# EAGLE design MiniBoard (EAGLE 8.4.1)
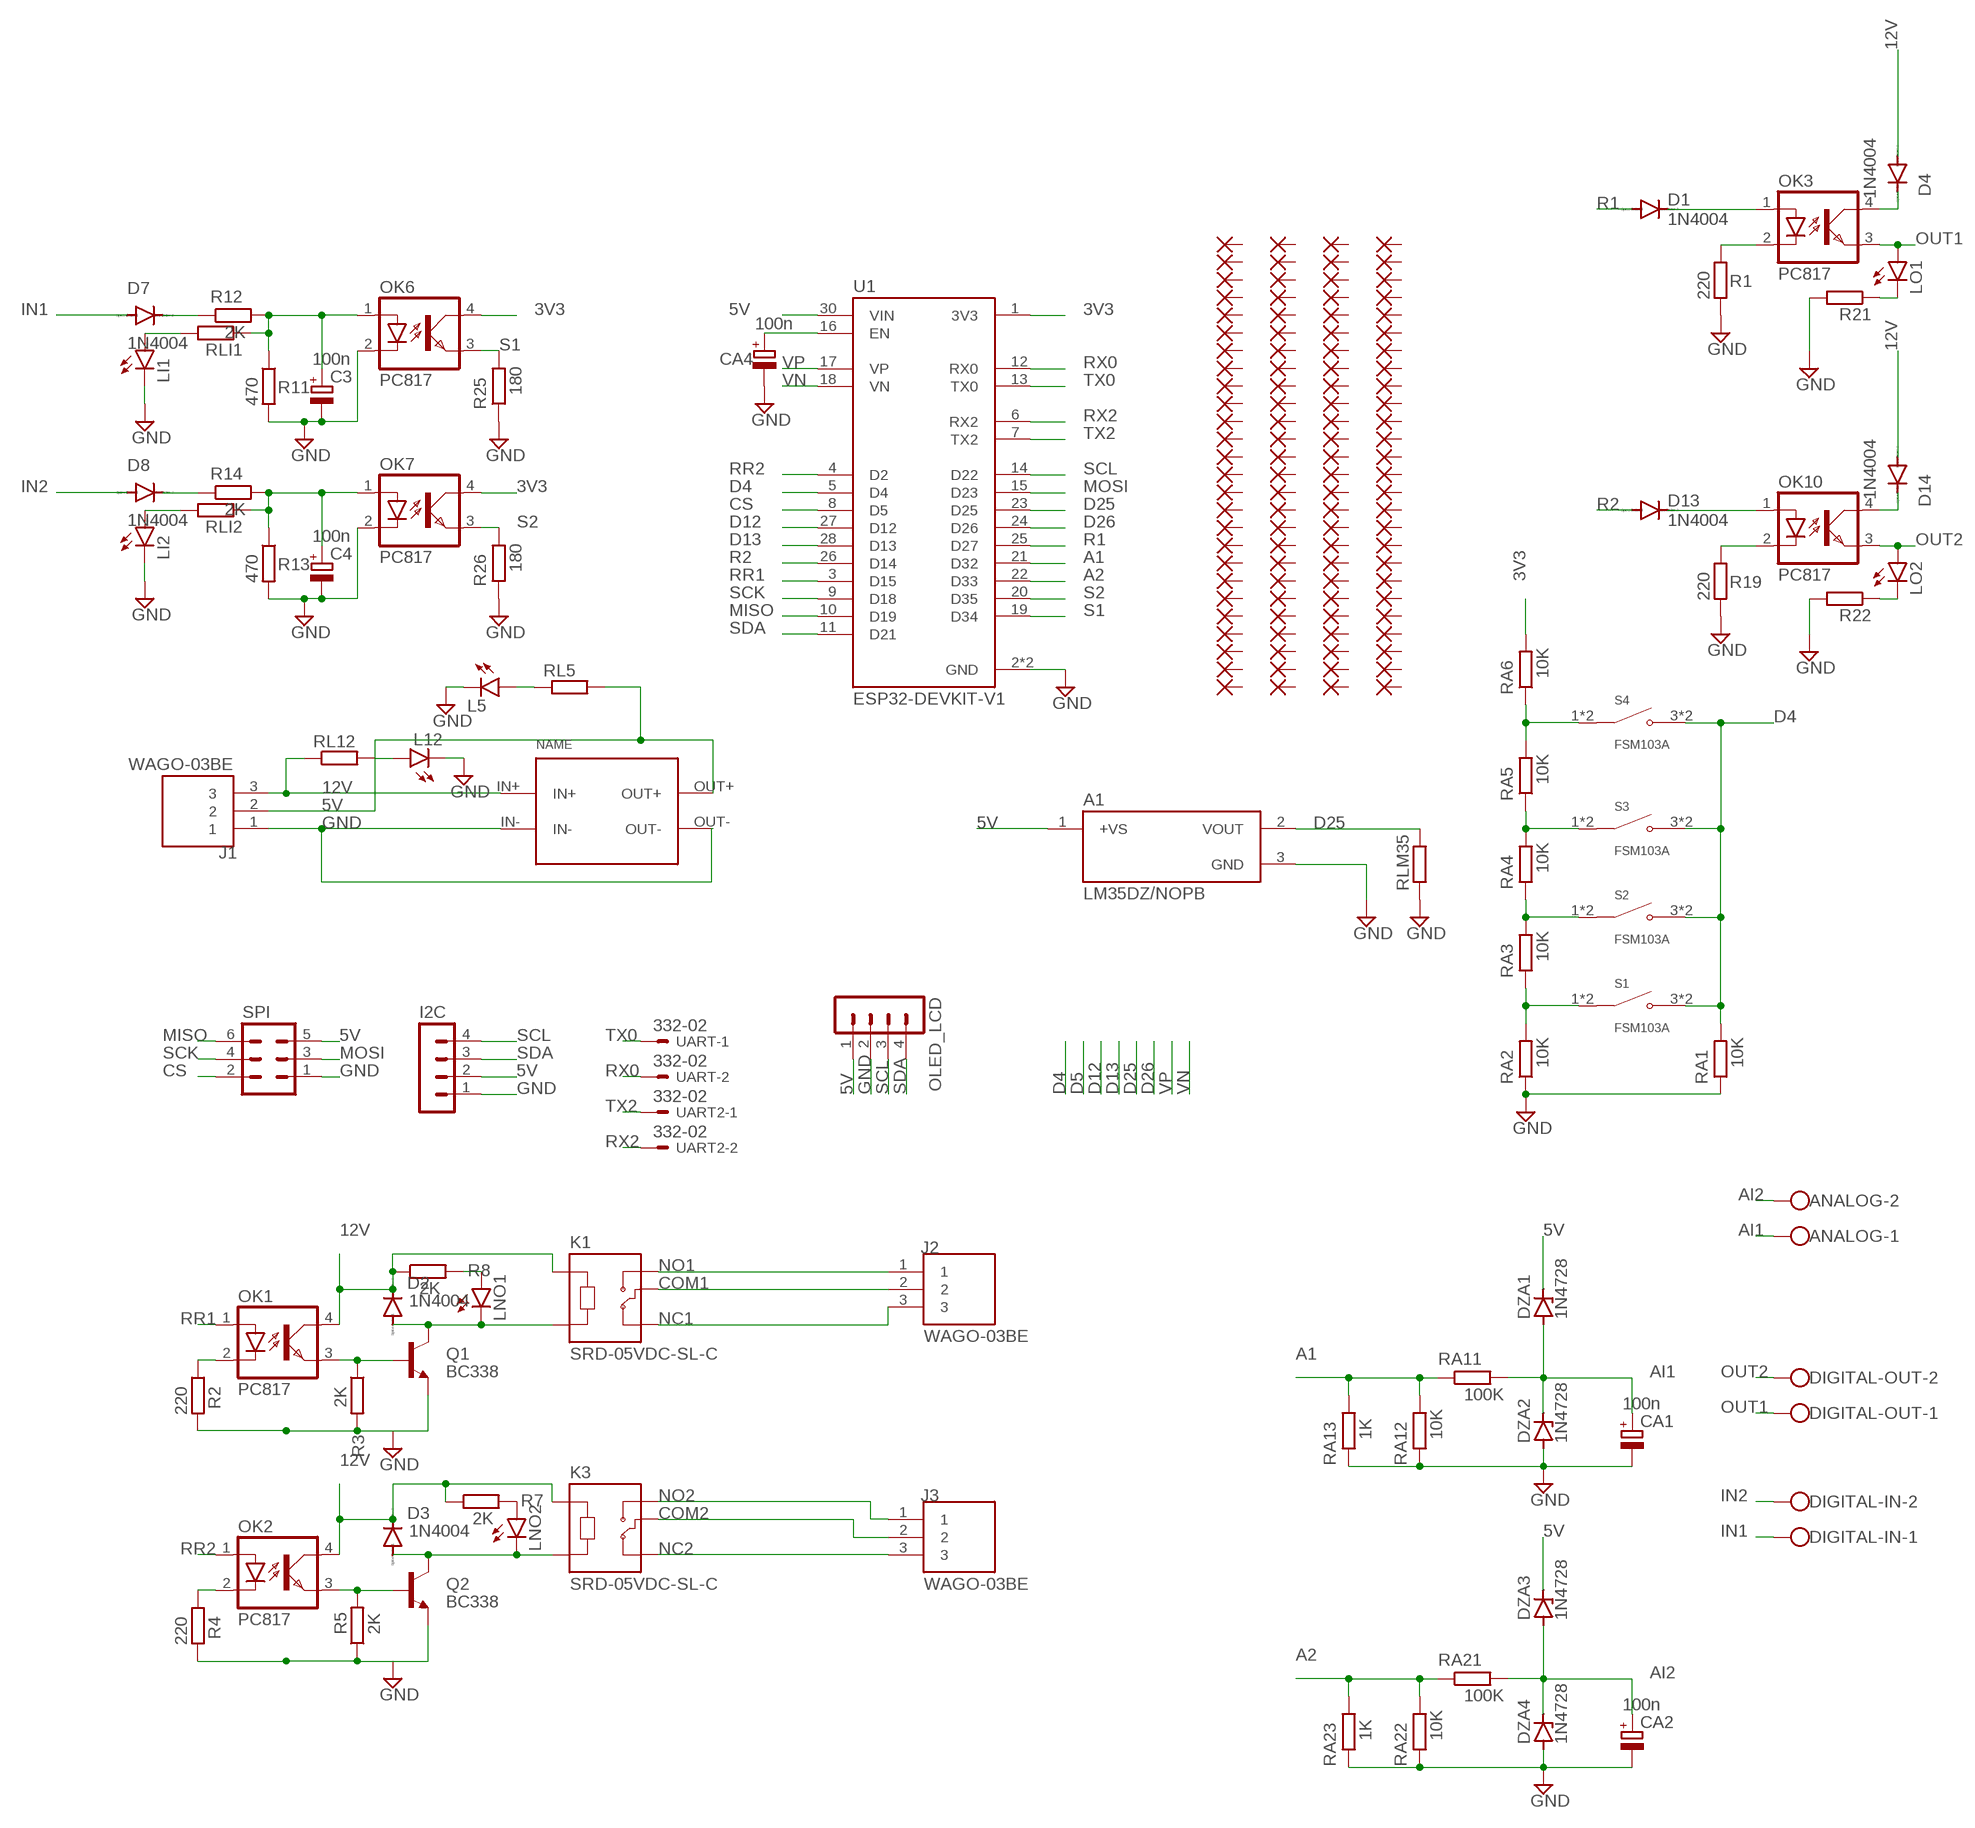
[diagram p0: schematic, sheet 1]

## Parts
A1  LM35DZ/NOPB  [TO92127P521H735-3]
ANALOG  W237-102  [W237-102]
C3  100n  CPOL-EUE5-6  [E5-6]
C4  100n  CPOL-EUE5-6  [E5-6]
CA1  100n  CPOL-EUE5-6  [E5-6]
CA2  100n  CPOL-EUE5-6  [E5-6]
CA4  100n  CPOL-EUE5-6  [E5-6]
D1  1N4004  [DO41-10]
D2  1N4004  [DO41-10]
D3  1N4004  [DO41-10]
D4  1N4004  [DO41-10]
D7  1N4004  [DO41-10]
D8  1N4004  [DO41-10]
D13  1N4004  [DO41-10]
D14  1N4004  [DO41-10]
DIGITAL-IN  W237-102  [W237-102]
DIGITAL-OUT  W237-102  [W237-102]
DZA1  1N4728  [DO41Z10]
DZA2  1N4728  [DO41Z10]
DZA3  1N4728  [DO41Z10]
DZA4  1N4728  [DO41Z10]
I2C  MA04-1  [MA04-1]
J1  WAGO-03BE  [CUI_TB006-508-03BE]
J2  WAGO-03BE  [CUI_TB006-508-03BE]
J3  WAGO-03BE  [CUI_TB006-508-03BE]
K1  SRD-05VDC-SL-C  [RELAY_SRD-05VDC-SL-C]
K3  SRD-05VDC-SL-C  [RELAY_SRD-05VDC-SL-C]
L5  LED3MM  [LED3MM]
L12  LED3MM  [LED3MM]
LI1  LED3MM  [LED3MM]
LI2  LED3MM  [LED3MM]
LNO1  LED3MM  [LED3MM]
LNO2  LED3MM  [LED3MM]
LO1  LED3MM  [LED3MM]
LO2  LED3MM  [LED3MM]
OK1  PC817  [DIL04]
OK2  PC817  [DIL04]
OK3  PC817  [DIL04]
OK6  PC817  [DIL04]
OK7  PC817  [DIL04]
OK10  PC817  [DIL04]
OLED_LCD  MA04-1  [MA04-1]
PAD1  WIREPAD1,6/0,9  [1,6/0,9]
PAD2  WIREPAD1,6/0,9  [1,6/0,9]
PAD3  WIREPAD1,6/0,9  [1,6/0,9]
PAD4  WIREPAD1,6/0,9  [1,6/0,9]
PAD5  WIREPAD1,6/0,9  [1,6/0,9]
PAD6  WIREPAD1,6/0,9  [1,6/0,9]
PAD7  WIREPAD1,6/0,9  [1,6/0,9]
PAD8  WIREPAD1,6/0,9  [1,6/0,9]
PAD9  WIREPAD1,6/0,9  [1,6/0,9]
PAD10  WIREPAD1,6/0,9  [1,6/0,9]
PAD11  WIREPAD1,6/0,9  [1,6/0,9]
PAD12  WIREPAD1,6/0,9  [1,6/0,9]
PAD13  WIREPAD1,6/0,9  [1,6/0,9]
PAD14  WIREPAD1,6/0,9  [1,6/0,9]
PAD15  WIREPAD1,6/0,9  [1,6/0,9]
PAD16  WIREPAD1,6/0,9  [1,6/0,9]
PAD17  WIREPAD1,6/0,9  [1,6/0,9]
PAD18  WIREPAD1,6/0,9  [1,6/0,9]
PAD19  WIREPAD1,6/0,9  [1,6/0,9]
PAD20  WIREPAD1,6/0,9  [1,6/0,9]
PAD21  WIREPAD1,6/0,9  [1,6/0,9]
PAD22  WIREPAD1,6/0,9  [1,6/0,9]
PAD23  WIREPAD1,6/0,9  [1,6/0,9]
PAD24  WIREPAD1,6/0,9  [1,6/0,9]
PAD25  WIREPAD1,6/0,9  [1,6/0,9]
PAD26  WIREPAD1,6/0,9  [1,6/0,9]
PAD27  WIREPAD1,6/0,9  [1,6/0,9]
PAD28  WIREPAD1,6/0,9  [1,6/0,9]
PAD29  WIREPAD1,6/0,9  [1,6/0,9]
PAD30  WIREPAD1,6/0,9  [1,6/0,9]
PAD31  WIREPAD1,6/0,9  [1,6/0,9]
PAD32  WIREPAD1,6/0,9  [1,6/0,9]
PAD33  WIREPAD1,6/0,9  [1,6/0,9]
PAD34  WIREPAD1,6/0,9  [1,6/0,9]
PAD35  WIREPAD1,6/0,9  [1,6/0,9]
PAD36  WIREPAD1,6/0,9  [1,6/0,9]
PAD37  WIREPAD1,6/0,9  [1,6/0,9]
PAD38  WIREPAD1,6/0,9  [1,6/0,9]
PAD39  WIREPAD1,6/0,9  [1,6/0,9]
PAD40  WIREPAD1,6/0,9  [1,6/0,9]
PAD41  WIREPAD1,6/0,9  [1,6/0,9]
PAD42  WIREPAD1,6/0,9  [1,6/0,9]
PAD43  WIREPAD1,6/0,9  [1,6/0,9]
PAD44  WIREPAD1,6/0,9  [1,6/0,9]
PAD45  WIREPAD1,6/0,9  [1,6/0,9]
PAD46  WIREPAD1,6/0,9  [1,6/0,9]
PAD47  WIREPAD1,6/0,9  [1,6/0,9]
PAD48  WIREPAD1,6/0,9  [1,6/0,9]
PAD49  WIREPAD1,6/0,9  [1,6/0,9]
PAD50  WIREPAD1,6/0,9  [1,6/0,9]
PAD51  WIREPAD1,6/0,9  [1,6/0,9]
PAD52  WIREPAD1,6/0,9  [1,6/0,9]
PAD53  WIREPAD1,6/0,9  [1,6/0,9]
PAD54  WIREPAD1,6/0,9  [1,6/0,9]
PAD55  WIREPAD1,6/0,9  [1,6/0,9]
PAD56  WIREPAD1,6/0,9  [1,6/0,9]
PAD57  WIREPAD1,6/0,9  [1,6/0,9]
PAD58  WIREPAD1,6/0,9  [1,6/0,9]
PAD59  WIREPAD1,6/0,9  [1,6/0,9]
PAD60  WIREPAD1,6/0,9  [1,6/0,9]
PAD61  WIREPAD1,6/0,9  [1,6/0,9]
PAD62  WIREPAD1,6/0,9  [1,6/0,9]
PAD63  WIREPAD1,6/0,9  [1,6/0,9]
PAD64  WIREPAD1,6/0,9  [1,6/0,9]
PAD65  WIREPAD1,6/0,9  [1,6/0,9]
PAD66  WIREPAD1,6/0,9  [1,6/0,9]
PAD67  WIREPAD1,6/0,9  [1,6/0,9]
PAD68  WIREPAD1,6/0,9  [1,6/0,9]
PAD69  WIREPAD1,6/0,9  [1,6/0,9]
PAD70  WIREPAD1,6/0,9  [1,6/0,9]
PAD71  WIREPAD1,6/0,9  [1,6/0,9]
PAD72  WIREPAD1,6/0,9  [1,6/0,9]
PAD73  WIREPAD1,6/0,9  [1,6/0,9]
PAD74  WIREPAD1,6/0,9  [1,6/0,9]
PAD75  WIREPAD1,6/0,9  [1,6/0,9]
PAD76  WIREPAD1,6/0,9  [1,6/0,9]
PAD77  WIREPAD1,6/0,9  [1,6/0,9]
PAD78  WIREPAD1,6/0,9  [1,6/0,9]
PAD79  WIREPAD1,6/0,9  [1,6/0,9]
PAD80  WIREPAD1,6/0,9  [1,6/0,9]
PAD81  WIREPAD1,6/0,9  [1,6/0,9]
PAD82  WIREPAD1,6/0,9  [1,6/0,9]
PAD83  WIREPAD1,6/0,9  [1,6/0,9]
PAD84  WIREPAD1,6/0,9  [1,6/0,9]
PAD85  WIREPAD1,6/0,9  [1,6/0,9]
PAD86  WIREPAD1,6/0,9  [1,6/0,9]
PAD87  WIREPAD1,6/0,9  [1,6/0,9]
PAD88  WIREPAD1,6/0,9  [1,6/0,9]
PAD89  WIREPAD1,6/0,9  [1,6/0,9]
PAD90  WIREPAD1,6/0,9  [1,6/0,9]
PAD91  WIREPAD1,6/0,9  [1,6/0,9]
PAD92  WIREPAD1,6/0,9  [1,6/0,9]
PAD93  WIREPAD1,6/0,9  [1,6/0,9]
PAD94  WIREPAD1,6/0,9  [1,6/0,9]
PAD95  WIREPAD1,6/0,9  [1,6/0,9]
PAD96  WIREPAD1,6/0,9  [1,6/0,9]
PAD97  WIREPAD1,6/0,9  [1,6/0,9]
PAD98  WIREPAD1,6/0,9  [1,6/0,9]
PAD99  WIREPAD1,6/0,9  [1,6/0,9]
PAD100  WIREPAD1,6/0,9  [1,6/0,9]
PAD101  WIREPAD1,6/0,9  [1,6/0,9]
PAD102  WIREPAD1,6/0,9  [1,6/0,9]
PAD103  WIREPAD1,6/0,9  [1,6/0,9]
PAD104  WIREPAD1,6/0,9  [1,6/0,9]
Q1  BC338  [TO92-EBC]
Q2  BC338  [TO92-EBC]
R1  220  R-EU_0309/12  [0309/12]
R2  220  R-EU_0309/12  [0309/12]
R3  2K  R-EU_0309/12  [0309/12]
R4  220  R-EU_0309/12  [0309/12]
R5  2K  R-EU_0309/12  [0309/12]
R7  2K  R-EU_0309/12  [0309/12]
R8  2K  R-EU_0309/12  [0309/12]
R11  470  R-EU_0309/12  [0309/12]
R12  2K  R-EU_0309/12  [0309/12]
R13  470  R-EU_0309/12  [0309/12]
R14  2K  R-EU_0309/12  [0309/12]
R19  220  R-EU_0309/12  [0309/12]
R21  R-EU_0309/12  [0309/12]
R22  R-EU_0309/12  [0309/12]
R25  180  R-EU_0309/12  [0309/12]
R26  180  R-EU_0309/12  [0309/12]
RA1  10K  R-EU_0309/12  [0309/12]
RA2  10K  R-EU_0309/12  [0309/12]
RA3  10K  R-EU_0309/12  [0309/12]
RA4  10K  R-EU_0309/12  [0309/12]
RA5  10K  R-EU_0309/12  [0309/12]
RA6  10K  R-EU_0309/12  [0309/12]
RA11  100K  R-EU_0309/12  [0309/12]
RA12  10K  R-EU_0309/12  [0309/12]
RA13  1K  R-EU_0309/12  [0309/12]
RA21  100K  R-EU_0309/12  [0309/12]
RA22  10K  R-EU_0309/12  [0309/12]
RA23  1K  R-EU_0309/12  [0309/12]
RL5  R-EU_0309/12  [0309/12]
RL12  R-EU_0309/12  [0309/12]
RLI1  R-EU_0309/12  [0309/12]
RLI2  R-EU_0309/12  [0309/12]
RLM35  R-EU_0309/12  [0309/12]
S1  FSM103A  [SW_1571627-1]
S2  FSM103A  [SW_1571627-1]
S3  FSM103A  [SW_1571627-1]
S4  FSM103A  [SW_1571627-1]
SPI  MA03-2  [MA03-2]
U1  ESP32-DEVKIT-V1  [MODULE_ESP32_DEVKIT_V1]
U$1  CP8-ADJ  [CP8-ADJ]
UART  332-02  [332-02]
UART2  332-02  [332-02]

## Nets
3V3: OK6.4(COL) OK7.4(COL) RA6.2 U1.1(3V3)
5V: A1.1(+VS) DZA1.C DZA3.C I2C.2 J1.2 OLED_LCD.1 RL5.2 SPI.5 U1.30(VIN) U$1.OUT+
12V: D2.C D3.C D4.A D14.A J1.3 K1.A1 K3.A1 OK1.4(COL) OK2.4(COL) R7.1 R8.1 RL12.1 U$1.IN+
A1: RA11.1 RA12.2 RA13.2 U1.21(D32)
A2: RA21.1 RA22.2 RA23.2 U1.22(D33)
AI1: ANALOG.1 CA1.+ DZA1.A DZA2.C RA11.2
AI2: ANALOG.2 CA2.+ DZA3.A DZA4.C RA21.2
COM1: J2.2 K1.COM
COM2: J3.2 K3.COM
CS: SPI.2 U1.8(D5)
D4: RA1.2 S1.3(NO) S1.4(NO) S2.3(NO) S2.4(NO) S3.3(NO) S3.4(NO) S4.3(NO) S4.4(NO) U1.5(D4)
D12: U1.27(D12)
D13: U1.28(D13)
D25: A1.2(VOUT) RLM35.2 U1.23(D25)
D26: U1.24(D26)
GND: A1.3(GND) C3.- C4.- CA1.- CA2.- CA4.- DZA2.A DZA4.A I2C.1 J1.1 L5.K(C) L12.K(C) LI1.K(C) LI2.K(C) OK6.2(C) OK7.2(C) OLED_LCD.2 Q1.E Q2.E R1.2 R2.2 R3.2 R4.2 R5.1 R11.2 R13.2 R19.2 R21.2 R22.2 R25.1 R26.1 RA1.1 RA2.1 RA12.1 RA13.1 RA22.1 RA23.1 RLM35.1 SPI.1 U1.2(GND) U1.29(GND) U$1.IN- U$1.OUT-
IN1: D7.A DIGITAL-IN.1
IN2: D8.A DIGITAL-IN.2
MISO: SPI.6 U1.10(D19)
MOSI: SPI.3 U1.15(D23)
N$1: OK2.2(C) R4.1
N$2: OK1.2(C) R2.1
N$3: OK1.3(EMIT) Q1.B R3.1
N$4: D3.A K3.A2 LNO2.K(C) Q2.C
N$5: RA4.2 RA5.1 S3.1(COM) S3.2(COM)
N$6: OK2.3(EMIT) Q2.B R5.2
N$7: LNO2.A R7.2
N$8: RA3.2 RA4.1 S2.1(COM) S2.2(COM)
N$9: RA2.2 RA3.1 S1.1(COM) S1.2(COM)
N$10: LNO1.A R8.2
N$11: D2.A K1.A2 LNO1.K(C) Q1.C
N$14: L12.A RL12.2
N$15: D1.C OK3.1(A)
N$16: OK3.2(C) R1.1
N$18: D4.C OK3.4(COL)
N$19: C3.+ OK6.1(A) R11.1 R12.2 RLI1.1
N$20: D7.C R12.1
N$21: C4.+ OK7.1(A) R13.1 R14.2 RLI2.1
N$22: D8.C R14.1
N$23: L5.A RL5.1
N$24: LI2.A RLI2.2
N$25: CA4.+ U1.16(EN)
N$26: D13.C OK10.1(A)
N$27: OK10.2(C) R19.1
N$29: LI1.A RLI1.2
N$30: LO1.K(C) R21.1
N$31: LO2.K(C) R22.1
N$32: RA5.2 RA6.1 S4.1(COM) S4.2(COM)
N$52: D14.C OK10.4(COL)
NC1: J2.3 K1.NC
NC2: J3.3 K3.NC
NO1: J2.1 K1.NO
NO2: J3.1 K3.NO
OUT1: DIGITAL-OUT.1 LO1.A OK3.3(EMIT)
OUT2: DIGITAL-OUT.2 LO2.A OK10.3(EMIT)
R1: D1.A U1.25(D27)
R2: D13.A U1.26(D14)
RR1: OK1.1(A) U1.3(D15)
RR2: OK2.1(A) U1.4(D2)
RX0: U1.12(RX0) UART.2
RX2: U1.6(RX2) UART2.2
S1: OK6.3(EMIT) R25.2 U1.19(D34)
S2: OK7.3(EMIT) R26.2 U1.20(D35)
SCK: SPI.4 U1.9(D18)
SCL: I2C.4 OLED_LCD.3 U1.14(D22)
SDA: I2C.3 OLED_LCD.4 U1.11(D21)
TX0: U1.13(TX0) UART.1
TX2: U1.7(TX2) UART2.1
VN: U1.18(VN)
VP: U1.17(VP)
Unconnected: PAD1.1(P) PAD2.1(P) PAD3.1(P) PAD4.1(P) PAD5.1(P) PAD6.1(P) PAD7.1(P) PAD8.1(P) PAD9.1(P) PAD10.1(P) PAD11.1(P) PAD12.1(P) PAD13.1(P) PAD14.1(P) PAD15.1(P) PAD16.1(P) PAD17.1(P) PAD18.1(P) PAD19.1(P) PAD20.1(P) PAD21.1(P) PAD22.1(P) PAD23.1(P) PAD24.1(P) PAD25.1(P) PAD26.1(P) PAD27.1(P) PAD28.1(P) PAD29.1(P) PAD30.1(P) PAD31.1(P) PAD32.1(P) PAD33.1(P) PAD34.1(P) PAD35.1(P) PAD36.1(P) PAD37.1(P) PAD38.1(P) PAD39.1(P) PAD40.1(P) PAD41.1(P) PAD42.1(P) PAD43.1(P) PAD44.1(P) PAD45.1(P) PAD46.1(P) PAD47.1(P) PAD48.1(P) PAD49.1(P) PAD50.1(P) PAD51.1(P) PAD52.1(P) PAD53.1(P) PAD54.1(P) PAD55.1(P) PAD56.1(P) PAD57.1(P) PAD58.1(P) PAD59.1(P) PAD60.1(P) PAD61.1(P) PAD62.1(P) PAD63.1(P) PAD64.1(P) PAD65.1(P) PAD66.1(P) PAD67.1(P) PAD68.1(P) PAD69.1(P) PAD70.1(P) PAD71.1(P) PAD72.1(P) PAD73.1(P) PAD74.1(P) PAD75.1(P) PAD76.1(P) PAD77.1(P) PAD78.1(P) PAD79.1(P) PAD80.1(P) PAD81.1(P) PAD82.1(P) PAD83.1(P) PAD84.1(P) PAD85.1(P) PAD86.1(P) PAD87.1(P) PAD88.1(P) PAD89.1(P) PAD90.1(P) PAD91.1(P) PAD92.1(P) PAD93.1(P) PAD94.1(P) PAD95.1(P) PAD96.1(P) PAD97.1(P) PAD98.1(P) PAD99.1(P) PAD100.1(P) PAD101.1(P) PAD102.1(P) PAD103.1(P) PAD104.1(P)

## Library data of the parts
A1 = LM35DZ_NOPB:LM35DZ/NOPB; CHECK_PRICES: https://www.snapeda.com/parts/LM35DZ/NOPB/Texas+Instruments/view-part/?ref=eda; DESCRIPTION: 1C high voltage analog temperature sensor, 10 mV/C; DIGIKEY_PART_NUMBER: LM35DZ/NOPB-ND; MF: Texas; MP: LM35DZ/NOPB; PACKAGE: None; SNAPEDA_LINK: https://www.snapeda.com/parts/LM35DZ/NOPB/Texas+Instruments/view-part/?ref=snap
ANALOG DIGITAL-IN DIGITAL-OUT = con-wago-500:W237-102: WAGO SCREW CLAMP; MPN: 237-102; OC_FARNELL: unknown; OC_NEWARK: 70K9898
C3 C4 CA1 CA2 CA4 = rcl-ws:CPOL-EU: POLARIZED CAPACITOR, European symbol; SPICEPREFIX: C
D1-D4 D7 D8 D13 D14 = diode:1N4004: DIODE
DZA1-DZA4 = diode-ws:1N4728: Z DIODE
I2C OLED_LCD = con-lstb:MA04-1: PIN HEADER; OC_FARNELL: unknown; OC_NEWARK: unknown
J1-J3 = TB006-508-03BE:WAGO-03BE: Check availability; AVAILABILITY: In Stock; CHECK_PRICES: https://www.snapeda.com/parts/TB006-508-03BE/Same+Sky/view-part/?ref=eda; DESCRIPTION: 2~24 Poles, Screw Type, Horizontal, 5.08 Pitch, 26~14 (AWG), Terminal Block Connector; MF: Same Sky; MP: TB006-508-03BE; PACKAGE: None; PRICE: None; SNAPEDA_LINK: https://www.snapeda.com/parts/TB006-508-03BE/Same+Sky/view-part/?ref=snap
K1 K3 = SRD-05VDC-SL-C:SRD-05VDC-SL-C: 5V Trigger Relay Module For Arduino And Raspberry Pi 5V Trigger Relay Module For Arduino And Raspberry Pi Check availability; AVAILABILITY: In Stock; CHECK_PRICES: https://www.snapeda.com/parts/SRD-05VDC-SL-C/Songle+Relay/view-part/?ref=eda; DESCRIPTION: 5V Trigger Relay Module For Arduino And Raspberry Pi 5V Trigger Relay Module For Arduino And Raspberry Pi; MF: Songle Relay; MP: SRD-05VDC-SL-C; PACKAGE: NON STANDARD-5 Songle Relay; PRICE: None; SNAPEDA_LINK: https://www.snapeda.com/parts/SRD-05VDC-SL-C/Songle+Relay/view-part/?ref=snap
L5 L12 LI1 LI2 LNO1 LNO2 LO1 LO2 = led_WS:LED: LED
OK1-OK3 OK6 OK7 OK10 = optocoupler:PC817: SHARP OPTO COUPLER; MPN: PC817X4J000F; OC_FARNELL: 9707727; OC_NEWARK: 97K7059
PAD1-PAD104 = wirepad-ws:WIREPAD: Wire PAD connect wire on PCB
Q1 Q2 = transistor-npn:BC338*: NPN Transistor
R1-R5 R7 R8 R11-R14 R19 R21 R22 R25 R26 RA1-RA6 RA11-RA13 RA21-RA23 RL5 RL12 RLI1 RLI2 RLM35 = rcl-ws:R-EU_: RESISTOR, European symbol; SPICEPREFIX: R
S1-S4 = FSM103A:FSM103A: Alcoswitch FSM100-104, Tactile Switches, Round Actuator Style, Operating Function NO, Brass Contact Base Material Check availability; AVAILABILITY: In Stock; CHECK_PRICES: https://www.snapeda.com/parts/FSM103A/TE+Connectivity+ALCOSWITCH+Switches/view-part/?ref=eda; COMMENT: 1571627-1; DESCRIPTION: Alcoswitch, Tactile switch,PCB,SPST,red actuator | TE Connectivity FSM103A; MF: TE Connectivity; MP: FSM103A; PACKAGE: None; PRICE: None; SNAPEDA_LINK: https://www.snapeda.com/parts/FSM103A/TE+Connectivity+ALCOSWITCH+Switches/view-part/?ref=snap
SPI = con-lstb-ws:MA03-2: PIN HEADER; OC_FARNELL: unknown; OC_NEWARK: unknown
U1 = ESP32-DEVKIT-V1:ESP32-DEVKIT-V1: Dual core, Wi-Fi: 2.4 GHz up to 150 Mbits/s,BLE (Bluetooth Low Energy) and legacy Bluetooth, 32 bits, Up to 240 MHz Check availability; AVAILABILITY: Not in stock; CHECK_PRICES: https://www.snapeda.com/parts/ESP32-DEVKIT-V1/Do+it/view-part/?ref=eda; DESCRIPTION: Dual core, Wi-Fi: 2.4 GHz up to 150 Mbits/s,BLE (Bluetooth Low Energy) and legacy Bluetooth, 32 bits, Up to 240 MHz; MF: Do it; MP: ESP32-DEVKIT-V1; PACKAGE: None; PRICE: None; SNAPEDA_LINK: https://www.snapeda.com/parts/ESP32-DEVKIT-V1/Do+it/view-part/?ref=snap
U$1 = userlib:CP8-ADJ: Voltage regulator IN: 7-35V OUT: ADJ
UART UART2 = con-garry-ws:332-02: 2 Pin - 2mm Dual Row

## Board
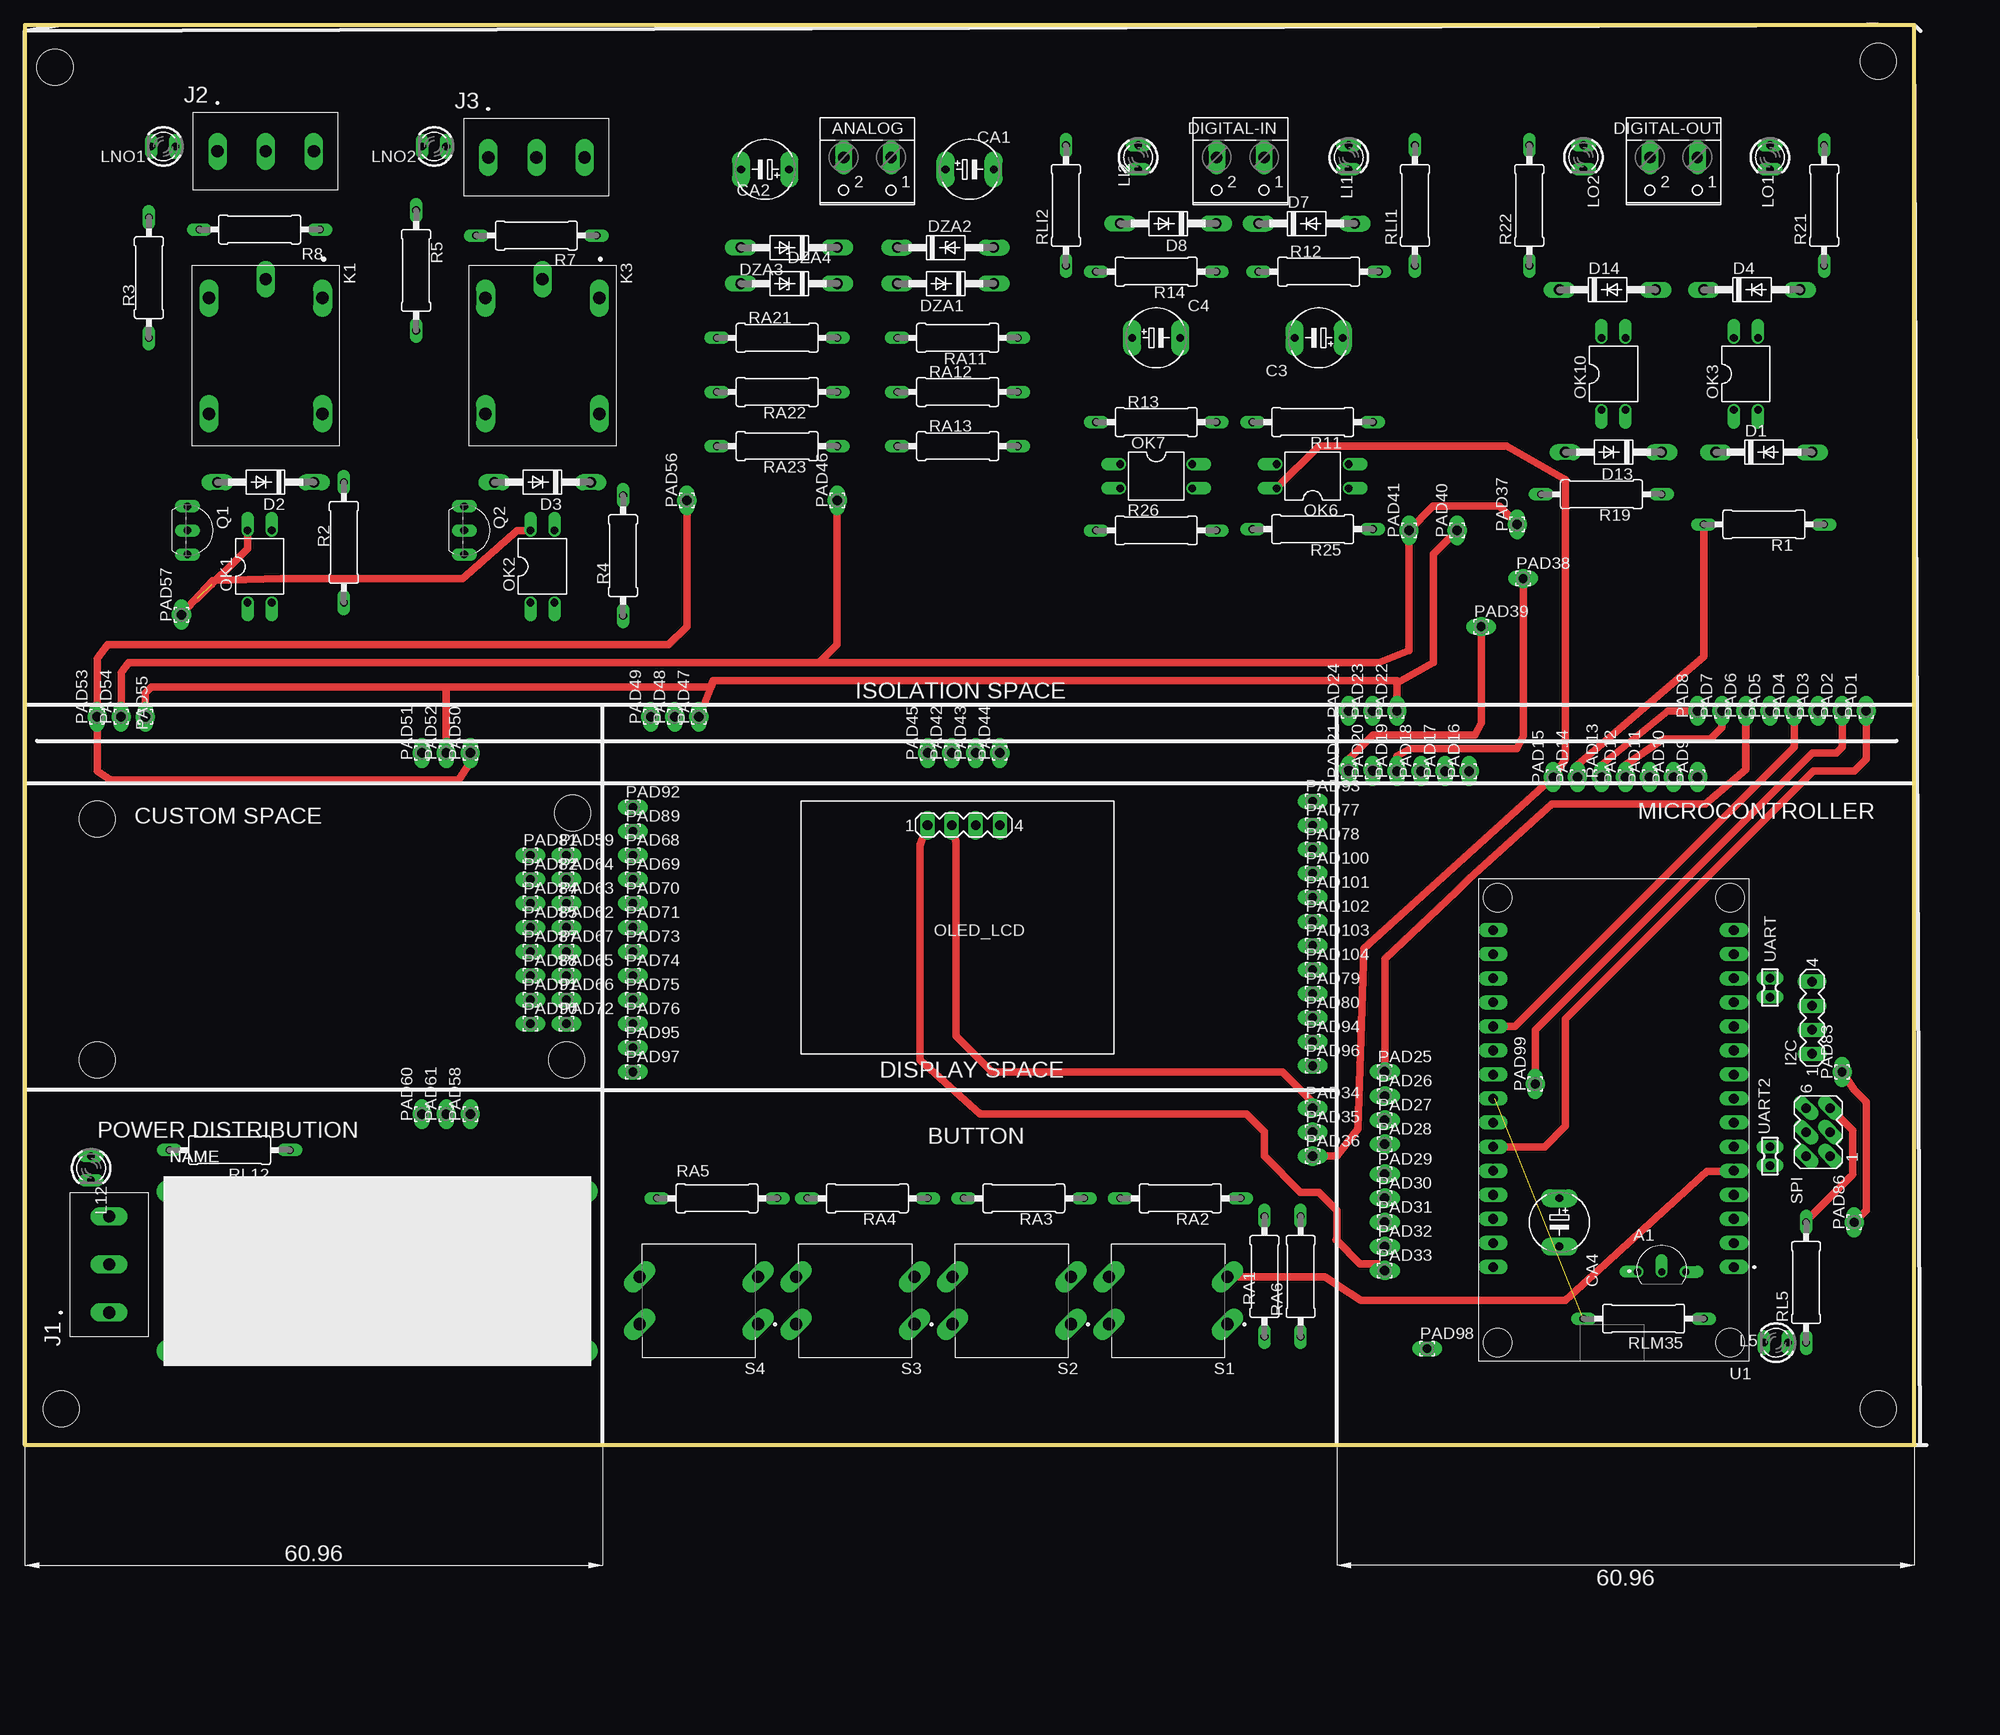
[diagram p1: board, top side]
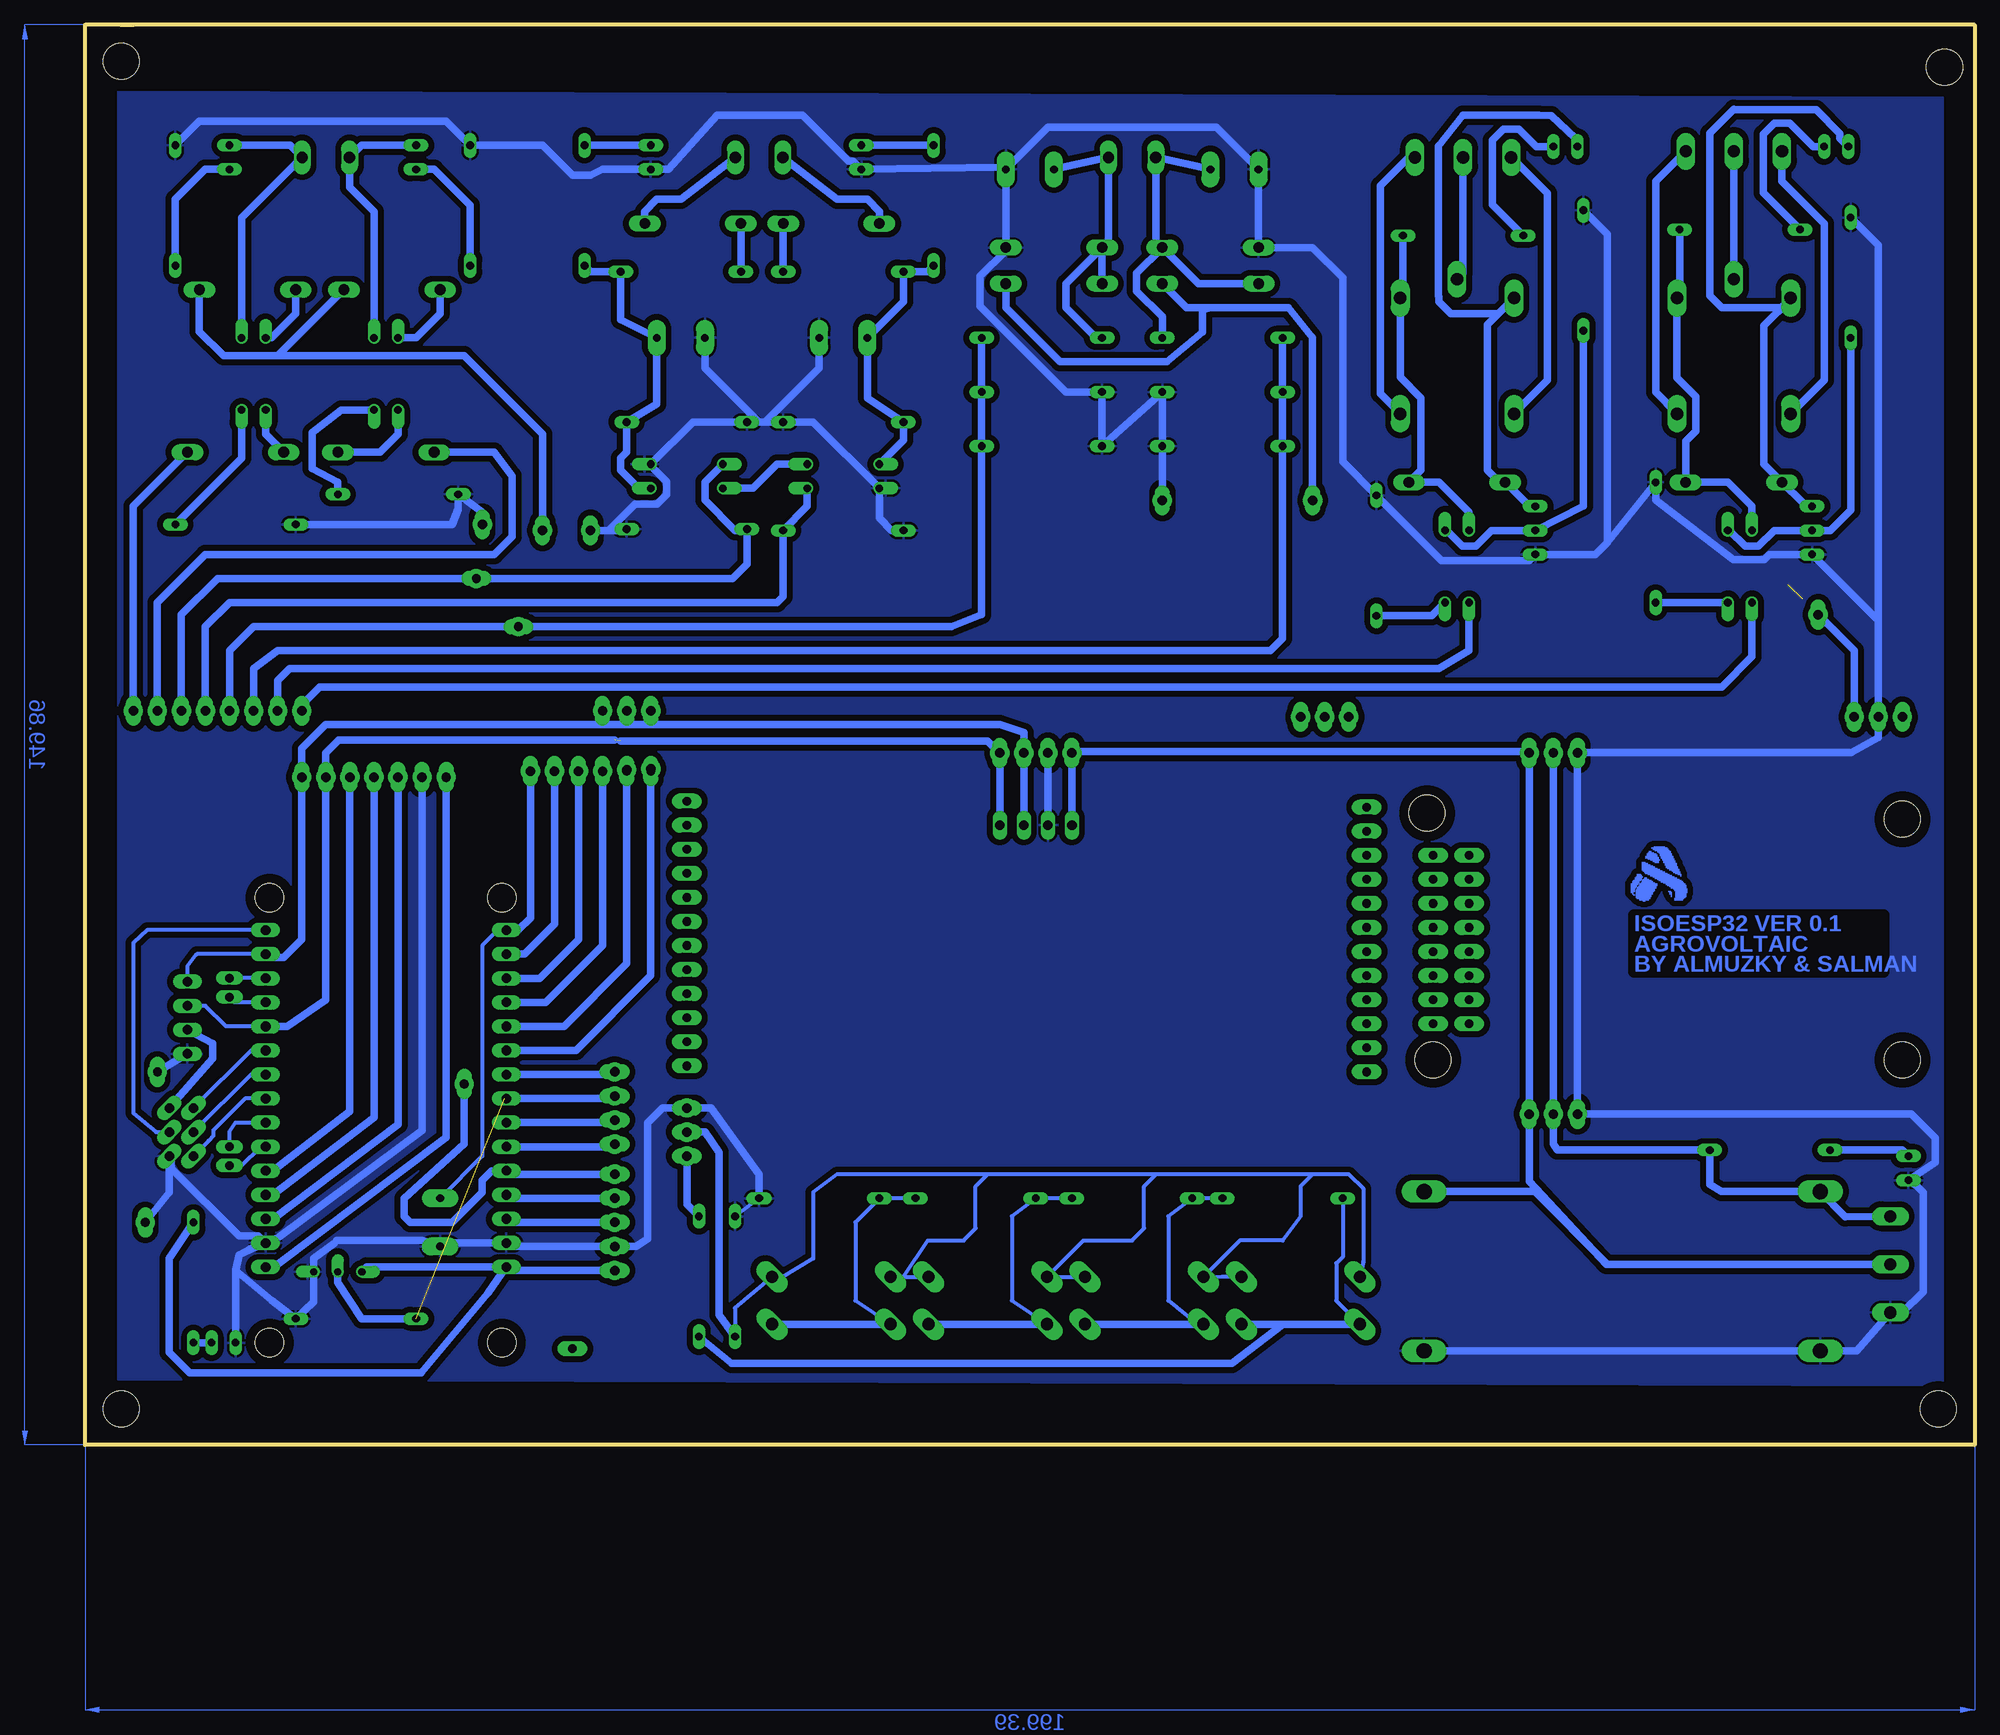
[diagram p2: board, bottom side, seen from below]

Size 199.39 x 149.86 mm. Coordinates in mm from the lower left corner, seen from the top.
Outline: 195.58,149.86 194.31,149.86
Outline: 0,0 199.39,0 199.39,149.86 0,149.86 0,0
Copper layers (1*16): Top 0.035mm / dielectric 1.5mm / Bottom 0.035mm
Design rules "default *": minimum track width 16mil, minimum drill 0.35mm, track to track 24mil, track to pad 24mil, pad to pad 24mil, via to via 6mil, smd to smd 6mil, copper to edge 40mil, drill to drill 6mil, minimum pad ring 10mil, minimum via ring 8mil, stop-mask expansion 4mil, vias tented up to drill 0mil, thermal gap 10mil
Holes 3.81 mm at 195.58,146.05 195.58,3.81 3.81,3.81 3.17,145.41 57.78,66.67 7.62,66.04 7.62,40.64 57.15,40.64

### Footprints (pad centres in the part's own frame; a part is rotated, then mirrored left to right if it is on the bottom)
TO92127P521H735-3 = drill 0.75 pad 0.813 offset: 1 -2.54,-0.775; 2 0,-0.775; 3 2.54,-0.775
W237-102 = drill 1.194 long: 1 -2.5,-1.27; 2 2.5,-1.27
E5-6 = drill 0.813 pad 1.905 long: + -2.54,0; - 2.54,0
DO41-10 = drill 1.118 long: A 5.08,0; C -5.08,0
DO41Z10 = drill 1.118 long: A 5.08,0; C -5.08,0
MA04-1 = drill 1.016 long: 1 -3.81,0; 2 -1.27,0; 3 1.27,0; 4 3.81,0
CUI_TB006-508-03BE = drill 1.3 long: 1 0,0; 2 5.08,0; 3 10.16,0
RELAY_SRD-05VDC-SL-C = drill 1.32 long: A1 -6.1,6; A2 -6.1,-6; NC 6.1,6; NO 6.1,-6 | drill 1.29 long: COM -8.1,0
LED3MM = drill 0.813 long: A -1.27,0; K 1.27,0
DIL04 = drill 0.813 offset: 1 -1.27,-3.81; 2 1.27,-3.81; 3 1.27,3.81; 4 -1.27,3.81
1,6/0,9 = drill 0.914 pad 1.6 long: 1 0,0
TO92-EBC = drill 0.813 long: B 0,-1.27; C -2.54,-1.27; E 2.54,-1.27
0309/12 = drill 0.813 long: 1 -6.35,0; 2 6.35,0
SW_1571627-1 = drill 1.3 long: 1 -6.25,2.5; 2 6.25,2.5; 3 -6.25,-2.5; 4 6.25,-2.5
MA03-2 = drill 1.016 pad 1.016 long: 1 -2.54,-1.27; 2 -2.54,1.27; 3 0,-1.27; 4 0,1.27; 5 2.54,-1.27; 6 2.54,1.27
MODULE_ESP32_DEVKIT_V1 = drill 1.02 pad 1.27 long: 1 -12.7,15.515; 2 -12.7,12.975; 3 -12.7,10.435; 4 -12.7,7.895; 5 -12.7,5.355; 6 -12.7,2.815; 7 -12.7,0.275; 8 -12.7,-2.265; 9 -12.7,-4.805; 10 -12.7,-7.345; 11 -12.7,-9.885; 12 -12.7,-12.425; 13 -12.7,-14.965; 14 -12.7,-17.505; 15 -12.7,-20.045; 16 12.7,-20.045; 17 12.7,-17.505; 18 12.7,-14.965; 19 12.7,-12.425; 20 12.7,-9.885; 21 12.7,-7.345; 22 12.7,-4.805; 23 12.7,-2.265; 24 12.7,0.275; 25 12.7,2.815; 26 12.7,5.355; 27 12.7,7.895; 28 12.7,10.435; 29 12.7,12.975; 30 12.7,15.515 | hole 3: -12.28,-23.475; 12.23,-23.475; 12.23,23.475; -12.28,23.475
CP8-ADJ = drill 1.6 long: IN+ -21.81,7.05; IN- -21.81,-9.75; OUT+ 19.99,7.05; OUT- 19.99,-9.75
332-02 = drill 0.9 pad 1.016 long: 1 0,-1; 2 0,1

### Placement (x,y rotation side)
A1  172.72,19.05 0 top
ANALOG  88.9,134.62 180 top
C3  136.53,116.84 180 top
C4  119.38,116.84 0 top
CA1  99.69,134.62 0 top
CA2  78.11,134.62 180 top
CA4  161.93,23.5 270 top
D1  183.51,104.78 0 top
D2  25.4,101.6 180 top
D3  54.61,101.6 180 top
D4  182.25,121.92 0 top
D7  135.25,128.91 0 top
D8  120.65,128.91 180 top
D13  167.64,104.78 180 top
D14  167,121.92 0 top
DIGITAL-IN  128.27,134.62 180 top
DIGITAL-OUT  173.99,134.62 180 top
DZA1  97.16,122.56 180 top
DZA2  97.16,126.36 0 top
DZA3  80.64,122.56 180 top
DZA4  80.64,126.36 180 top
I2C  188.59,45.09 90 top
J1  8.89,13.97 90 top
J2  20.32,136.53 0 top
J3  48.9,135.89 0 top
K1  25.4,114.94 270 top
K3  54.61,114.94 270 top
L5  184.78,10.79 180 top
L12  6.99,29.21 270 top
LI1  139.7,135.89 270 top
LI2  117.47,135.89 270 top
LNO1  14.61,137.03 180 top
LNO2  43.18,137.03 180 top
LO1  184.15,135.89 270 top
LO2  164.47,135.89 270 top
OK1  24.77,92.71 0 top
OK2  54.61,92.71 0 top
OK3  181.61,113.03 0 top
OK6  135.89,102.23 90 top
OK7  119.38,102.23 270 top
OK10  167.64,113.03 0 top
OLED_LCD  99.06,65.41 0 top
PAD1  194.31,77.47 90 top
PAD2  191.77,77.47 90 top
PAD3  189.23,77.47 90 top
PAD4  186.69,77.47 90 top
PAD5  184.15,77.47 90 top
PAD6  181.61,77.47 90 top
PAD7  179.07,77.47 90 top
PAD8  176.53,77.47 90 top
PAD9  176.53,70.48 90 top
PAD10  173.99,70.48 90 top
PAD11  171.45,70.48 90 top
PAD12  168.91,70.48 90 top
PAD13  166.37,70.48 90 top
PAD14  163.83,70.48 90 top
PAD15  161.29,70.48 90 top
PAD16  152.4,71.12 90 top
PAD17  149.86,71.12 90 top
PAD18  147.32,71.12 90 top
PAD19  144.78,71.12 90 top
PAD20  142.24,71.12 90 top
PAD21  139.7,71.12 90 top
PAD22  144.78,77.47 90 top
PAD23  142.24,77.47 90 top
PAD24  139.7,77.47 90 top
PAD25  143.51,39.37 0 top
PAD26  143.51,36.83 0 top
PAD27  143.51,34.29 0 top
PAD28  143.51,31.75 0 top
PAD29  143.51,28.57 0 top
PAD30  143.51,26.04 0 top
PAD31  143.51,23.5 0 top
PAD32  143.51,20.95 0 top
PAD33  143.51,18.41 0 top
PAD34  135.89,35.56 0 top
PAD35  135.89,33.02 0 top
PAD36  135.89,30.48 0 top
PAD37  157.48,97.16 90 top
PAD38  158.12,91.44 0 top
PAD39  153.67,86.36 0 top
PAD40  151.13,96.52 90 top
PAD41  146.05,96.52 90 top
PAD42  97.79,73.03 90 top
PAD43  100.33,73.03 90 top
PAD44  102.87,73.03 90 top
PAD45  95.25,73.03 90 top
PAD46  85.72,99.69 90 top
PAD47  71.12,76.83 90 top
PAD48  68.58,76.83 90 top
PAD49  66.04,76.83 90 top
PAD50  46.99,73.03 90 top
PAD51  41.91,73.03 90 top
PAD52  44.45,73.03 90 top
PAD53  7.62,76.83 90 top
PAD54  10.16,76.83 90 top
PAD55  12.7,76.83 90 top
PAD56  69.85,99.69 90 top
PAD57  16.51,87.63 90 top
PAD58  46.99,34.92 90 top
PAD59  57.15,62.23 0 top
PAD60  41.91,34.92 90 top
PAD61  44.45,34.92 90 top
PAD62  57.15,54.61 0 top
PAD63  57.15,57.15 0 top
PAD64  57.15,59.69 0 top
PAD65  57.15,49.53 0 top
PAD66  57.15,46.99 0 top
PAD67  57.15,52.07 0 top
PAD68  64.14,62.23 0 top
PAD69  64.14,59.69 0 top
PAD70  64.14,57.15 0 top
PAD71  64.14,54.61 0 top
PAD72  57.15,44.45 0 top
PAD73  64.14,52.07 0 top
PAD74  64.14,49.53 0 top
PAD75  64.14,46.99 0 top
PAD76  64.14,44.45 0 top
PAD77  135.89,65.41 0 top
PAD78  135.89,62.87 0 top
PAD79  135.89,47.62 0 top
PAD80  135.89,45.09 0 top
PAD81  53.34,62.23 0 top
PAD82  53.34,59.69 0 top
PAD83  191.77,39.37 90 top
PAD84  53.34,57.15 0 top
PAD85  53.34,54.61 0 top
PAD86  193.04,23.5 90 top
PAD87  53.34,52.07 0 top
PAD88  53.34,49.53 0 top
PAD89  64.14,64.77 0 top
PAD90  53.34,44.45 0 top
PAD91  53.34,46.99 0 top
PAD92  64.14,67.31 0 top
PAD93  135.89,67.94 0 top
PAD94  135.89,42.55 0 top
PAD95  64.14,41.91 0 top
PAD96  135.89,40.01 0 top
PAD97  64.14,39.37 0 top
PAD98  147.96,10.16 0 top
PAD99  159.38,38.1 90 top
PAD100  135.89,60.33 0 top
PAD101  135.89,57.78 0 top
PAD102  135.89,55.24 0 top
PAD103  135.89,52.7 0 top
PAD104  135.89,50.16 0 top
Q1  18.41,96.52 270 top
Q2  47.62,96.52 270 top
R1  183.51,97.16 180 top
R2  33.66,95.25 90 top
R3  13.08,123.19 90 top
R4  63.12,93.85 90 top
R5  41.27,123.95 270 top
R7  53.98,127.64 180 top
R8  24.77,128.27 180 top
R11  135.89,107.95 180 top
R12  136.53,123.83 0 top
R13  119.38,107.95 0 top
R14  119.38,123.83 180 top
R19  166.37,100.33 180 top
R21  189.87,130.81 90 top
R22  158.75,130.81 90 top
R25  135.89,96.65 180 top
R26  119.38,96.52 0 top
RA1  130.81,17.78 270 top
RA2  121.92,26.04 180 top
RA3  105.41,26.04 180 top
RA4  88.9,26.04 180 top
RA5  73.03,26.04 180 top
RA6  134.62,17.78 90 top
RA11  98.42,116.84 180 top
RA12  98.42,111.12 0 top
RA13  98.42,105.41 0 top
RA21  79.38,116.84 0 top
RA22  79.38,111.12 180 top
RA23  79.38,105.41 180 top
RL5  187.96,17.14 90 top
RL12  21.59,31.11 180 top
RLI1  146.69,130.81 90 top
RLI2  109.86,130.81 90 top
RLM35  170.81,13.34 180 top
S1  120.65,15.24 180 top
S2  104.14,15.24 180 top
S3  87.63,15.24 180 top
S4  71.12,15.24 180 top
SPI  189.23,33.02 90 top
U1  167.64,34.29 180 top
U$1  38.1,19.68 0 top
UART  184.15,48.26 180 top
UART2  184.15,30.48 180 top

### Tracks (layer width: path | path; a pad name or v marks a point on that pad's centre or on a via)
3V3  (via drill 1 pad 2.03)
  Top 0.813: v135.89,30.48 138.43,30.48 140.65,33.34 141.29,52.39 v161.29,70.48 | 161.13,70.8 v161.29,70.48 | OK6.4 136.53,105.41 156.37,105.41 162.56,101.87 162.56,72.39 v161.29,70.48
  Bottom 0.813: RA6.2 135.89,25.4 v135.89,30.48 | v161.29,70.48 161.29,32.46 179.42,18.77 U1.1 | OK7.4 126.36,103.5 128.91,100.97 OK6.4
5V  (via drill 1 pad 2.03)
  Top 0.813: OLED_LCD.1 94.46,63.34 94.46,40.64 100.81,34.92 128.91,34.92 130.81,33.02 130.81,30.48 134.62,26.67 136.53,26.67 138.43,24.77 138.43,21.59 | v46.99,73.03 46.99,72.01 45.78,70.17 9.04,70.17 7.62,71.1 v7.62,76.83 7.62,82.97 8.73,84.45 67.94,84.45 69.85,86.36 v69.85,99.69 | 138.35,21.67 138.43,21.59 | SPI.5 192.89,33.17 192.89,28.57 187.96,23.65 RL5.2 | 138.43,21.59 140.89,19.13 142.8,19.13 v143.51,18.41
  Bottom 0.406: 156.57,18.77 U1.30
  Bottom 0.813: I2C.2 185.9,42.39 185.9,40.79 SPI.5 | U$1.OUT+ 46.42,26.73 38.73,19.05 | J1.2 38.73,19.05 | 38.73,19.05 38.86,19.05 46.99,27.81 v46.99,34.92 v46.99,73.03 46.99,73.18 95.25,73.18 v95.25,73.03 OLED_LCD.1 | v69.85,99.69 69.85,116.84 72.39,120.02 80.64,120.02 | 143.51,18.14 v143.51,18.41 154.58,18.41 U1.30 | RL5.2 190.5,19.68 190.5,9.79 188.33,7.62 163.9,7.62 156.84,16.05 U1.30 | 169.41,18.14 A1.1 169.68,18.77 U1.30 | 80.64,120.02 83.19,120.02 DZA3.C | 80.64,120.02 81.48,119.81 81.48,117.42 85.23,114.3 96.52,114.3 102.23,120.02 DZA1.C
12V  (via drill 0.35, 1 pad 2.03)  (1 unrouted)
  Top 0.813: 72.39,80.01 46.35,80.01 44.45,80.01 | 44.45,80.01 13.34,80.01 12.7,79.38 v12.7,76.83 | 72.39,80.01 72.64,80.64 144.78,80.64 144.78,80.43 | 72.39,80.01 v71.12,76.83 | 151.13,95.89 v151.13,96.52 148.65,94.04 148.65,82.58 144.78,80.43 | 144.78,80.43 v144.78,77.47 | v16.51,87.63 19.79,91.2 | 19.79,91.2 19.68,90.81 | OK2.4 51.93,96.52 46.21,91.44 27.02,91.44 19.79,91.2 | OK1.4 23.5,94.61 18.19,89.31 | v44.45,73.03 44.45,80.01
  Bottom 0.813: J1.3 13.63,24.08 U$1.IN+ 26.75,26.73 27.94,27.52 RL12.1 44.03,31.11 44.45,31.75 v44.45,34.92 v44.45,73.03 | v151.13,96.52 151.13,106.68 159.38,114.94 179.07,114.94 | R7.1 60.33,121.32 K3.A1 60.61,112.68 58.42,110.49 58.42,102.87 D3.C 56.52,101.6 53.34,98.42 OK2.4 | R8.1 31.11,121.32 K1.A1 31.4,112.66 29.39,110.66 29.39,107.01 30.48,105.93 D2.C 26.04,101.6 23.5,99.06 OK1.4 | D14.A 179.07,114.94 | 179.07,114.94 184.78,114.94 187.32,117.47 D4.A | v16.51,87.63 12.7,83.82 v12.7,76.83
  other vias: 53.34,96.52
A1  (via drill 0.9 pad 2.03, 1 pad 2.03)
  Top 0.813: v139.7,71.37 139.7,72.39 142.24,74.93 153.03,74.93 153.67,76.2 v153.67,86.36
  Bottom 0.406: U1.21 154.94,41.91
  Bottom 0.813: RA11.1 RA12.2 RA13.2 104.78,87.63 107.95,86.36 v153.67,86.36 181.61,86.36 184.15,83.82 v184.15,77.47 | v139.7,71.37 139.7,49.53 147.59,41.63 U1.21
A2  (via drill 1 pad 2.03)
  Top 0.813: v143.51,39.37 143.51,51.28 151.05,58.44 151.72,59.1 152.36,59.74 161.13,67.63 177.32,67.63 181.61,71.28 v181.61,77.47
  Bottom 0.406: U1.22 154.94,38.73
  Bottom 0.813: RA21.1 RA22.2 RA23.2 73.03,85.09 74.3,83.82 179.07,83.82 181.61,81.92 v181.61,77.47 | U1.22 143.78,39.09 v143.51,39.37
AI1
  Bottom 0.813: DZA2.C DZA1.A | CA1.+ ANALOG.1 91.4,127.04 DZA2.C | DZA2.C 95.89,122.56 95.89,120.02 92.71,116.84 RA11.2
AI2
  Bottom 0.813: CA2.+ ANALOG.2 | ANALOG.2 86.4,134.03 | DZA3.A 81.92,122.56 DZA4.C | RA21.2 85.72,119.09 88.42,121.79 88.42,123.67 DZA4.C | ANALOG.2 86.4,127.04 DZA4.C
COM1
  Bottom 0.813: J2.2 K1.COM
COM2
  Bottom 0.813: J3.2 53.98,123.67 K3.COM
CS
  Bottom 0.406: U1.8 182.51,36.55 185.85,33.22 185.85,32.63 186.37,32.11 186.37,32.07 SPI.2
D4  (via drill 1 pad 2.03)
  Top 0.813: U1.5 179.71,28.89 177.48,28.89 162.56,15.24 140.97,15.24 137.2,17.74 S1.3
  Bottom 0.406: 81.97,17.78 S3.4 | S1.4 113.03,17.74 | 113.03,17.74 S2.3 | S3.3 S2.4 94.04,21.59 88.9,21.59 87.63,22.86 87.63,27.3 86.36,28.57 | S3.4 80.69,17.74 79.38,17.78 78.68,17.78 S4.3 | 69.85,28.57 66.04,28.57 64.52,27.05 64.52,19.36 S4.4 | 69.85,28.57 86.36,28.57 | 86.36,28.57 104.14,28.57 | 104.14,28.57 120.02,28.57 122.56,26.67 122.56,19.68 125.77,17.74 S1.3 130.81,14.46 RA1.2 | S3.4 77.53,21.59 73.03,21.59 71.12,24.13 71.12,27.3 69.85,28.57 | 113.03,17.74 110.45,21.59 106.68,21.59 105.41,22.86 105.41,27.3 104.14,28.57
  Bottom 0.813: RA1.2 132.49,13.74 132.49,30.89 133.99,33.02 v135.89,33.02 | v171.45,70.48 171.45,35.18 179.6,28.93 U1.5
D12  (via drill 1 pad 2.03)
  Bottom 0.406: U1.27 154.94,26.04
  Bottom 0.813: v143.51,26.04 154.94,26.04 155.22,26.67 U1.27
D13  (via drill 1 pad 2.03)
  Bottom 0.813: 143.51,23.22 v143.51,23.5 153.94,23.5 U1.28
D25  (via drill 1 pad 2.03)  (1 unrouted)
  Bottom 0.406: 155.12,36.55 U1.23
  Bottom 0.813: U1.23 143.51,36.55 v143.51,36.83 | RLM35.2 170.18,13.34 172.72,17.14 A1.2
D26  (via drill 1 pad 2.03)
  Bottom 0.813: U1.24 143.51,34.02 v143.51,34.29
GND  (via drill 0.9 pad 2.03, 1 pad 2.03)
  Top 0.813: v85.72,99.69 85.72,84.45 83.82,82.55 | v10.16,76.83 10.16,81.49 10.95,82.55 83.82,82.55 | 86.36,82.55 83.82,82.55 | 85.79,82.58 85.82,82.55 142.88,82.55 146.05,83.82 v146.05,96.52 148.59,99.06 155.57,99.06 v157.48,97.16 | OLED_LCD.2 98.27,63.66 98.27,43.18 102.08,39.37 132.72,39.37 135.89,36.2 v135.89,35.56 | R1.2 177.16,83.19 163.83,71.75 v163.83,70.48 | v191.77,39.37 193.04,37.47 194.31,36.2 194.31,24.77 v193.04,23.5
  Bottom 0.406: RA2.1 RA1.1
  Bottom 0.813: U$1.IN- 15.88,9.53 | L5.K 183.51,18.41 | 183.51,18.41 183.16,20.05 | 183.16,20.05 U1.2 | CA4.- 163.47,20.68 | U$1.OUT- U$1.IN- | U$1.IN- 12.44,9.94 J1.1 7.62,13.97 5.44,16.15 5.44,26.67 6.07,27.3 L12.K 4.17,29.84 4.17,32.38 6.71,34.92 v41.91,34.92 v41.91,73.03 41.15,73.09 13.02,73.09 10.16,74.68 v10.16,76.83 | RA2.1 128.27,28.57 133.35,35.56 v135.89,35.56 138.43,35.56 140.02,33.97 140.02,21.72 141.24,20.95 v143.51,20.95 | v85.72,99.69 RA23.1 RA22.1 RA13.1 RA12.1 95.89,111.12 104.93,120.17 104.93,123.32 102.23,126.02 DZA2.A CA1.- | 127.64,107.95 R13.2 122.56,107.95 OK7.2 115.57,97.79 114.3,96.52 R26.1 | 128.27,107.95 127.64,107.95 | 128.27,107.95 R11.2 135.25,107.95 OK6.2 139.7,103.34 138.02,101.66 138.02,100.27 139.01,99.29 141.38,99.29 144.15,96.52 | R1.2 160.66,97.16 160.02,98.74 R19.2 157.48,98.42 v157.48,97.16 | OLED_LCD.2 v97.79,73.03 | U1.2 181.97,20.68 | 181.97,20.68 178.89,21.95 163.83,33.2 v163.83,70.48 | 143.51,20.68 v143.51,20.95 | 144.15,96.52 v146.05,96.52 | 144.15,96.52 142.37,96.52 R25.1 | CA4.- 162.92,21.32 U1.29 154.58,20.95 v143.51,20.95 | 181.97,20.68 183.16,20.05 | I2C.1 v191.77,39.37 | v193.04,23.5 190.5,26.67 SPI.1 190.28,30.26 190.28,29.2 183.15,22.07 181.1,22.07 U1.2 | 183.51,18.41 179.71,15.24 RLM35.1 175.26,15.1 A1.3 175.26,19.68 173.13,21.29 172.82,21.59 163.83,21.59 CA4.- | 10.16,87 Q1.E 21.65,93.98 22.21,93.42 25.48,93.42 33.66,99.69 R2.2 38.73,95.25 | 10.16,87 10.16,76.91 | R3.2 10.16,126.62 10.16,87 | CA1.- 97.79,139.06 80.01,139.06 CA2.- DZA4.A 69.85,126.36 66.67,123.19 66.67,103.76 R4.2 56.26,93.34 46.99,93.34 Q2.E 40.01,93.98 38.73,95.25
  Bottom 0.813: CA1.- 102.56,134.62 102.78,134.84 LI2.K 118.34,135.48 118.83,135.48 123.68,140.34 132.72,140.34 137.79,134.62 LI1.K 144.78,134.62 146.05,133.99 147.96,133.99 151.13,137.16 R22.2 161.29,139.7 187.32,139.7 R21.2 | R5.1 38.73,127.76 38.73,95.25 | C4.- 121.92,113.67 127.64,107.95 | C3.- 133.99,113.67 128.27,107.95
  pour Bottom: 3.3,142.25 195.96,142.87 195.96,6.86 3.3,6.24
IN1
  Bottom 0.813: DIGITAL-IN.1 136.49,131.44 139.06,131.44 140.34,130.18 D7.A
IN2
  Bottom 0.813: DIGITAL-IN.2 120.06,131.44 116.84,131.44 115.57,130.18 D8.A
MISO
  Bottom 0.406: U1.10 181.88,41.63 SPI.6
MOSI
  Bottom 0.406: U1.15 192.84,54.34 194.31,52.99 194.31,35.03 191.9,33.02 SPI.3
N$1
  Bottom 0.813: R4.1 57.28,87.5 OK2.2
N$2
  Bottom 0.813: R2.1 OK1.2
N$3
  Bottom 0.813: R3.1 13.08,98.68 15.24,96.52 Q1.B 21.12,96.52 22.8,94.84 24.19,94.84 25.87,96.52 OK1.3
N$4
  Bottom 0.813: LNO2.K 42.14,137.9 44.68,140.29 45.99,140.34 53.98,140.34 56.59,137.08 56.59,121.25 56.52,121.17 56.52,120.65 55.24,119.38 50.27,119.38 | K3.A2 50.27,119.38 | 50.27,119.38 51.44,118.21 51.44,102.87 50.16,101.6 D3.A 46.99,99.06 Q2.C
N$5
  Bottom 0.406: RA5.1 RA4.2 85.09,24.13 85.09,15.24 81.95,12.74
  Bottom 0.813: S3.2 81.95,12.74 S3.1
N$6
  Bottom 0.813: R5.2 41.27,99.06 Q2.B 50.97,96.52 52.65,94.84 54.03,94.84 55.71,96.52 OK2.3
N$7
  Bottom 0.813: LNO2.A 46.25,137.03 48.07,138.86 49.72,138.86 50.89,137.69 50.89,130.9 R7.2
N$8
  Bottom 0.406: RA4.1 RA3.2 101.6,24.13 101.6,15.24 97.83,12.74
  Bottom 0.813: 97.83,12.74 S2.2 S2.1
N$9
  Bottom 0.406: RA3.1 RA2.2 118.11,23.5 118.11,15.24 114.34,12.74
  Bottom 0.813: 114.34,12.74 S1.2 S1.1 126.94,12.7 127,12.7
N$10
  Bottom 0.813: LNO1.A 17.04,137.03 19.5,139.49 21.14,139.49 22.31,138.32 22.31,132.17 R8.2
N$11
  Bottom 0.813: LNO1.K 14.2,137.9 14.2,138.39 16.72,140.91 25.34,140.91 25.4,140.97 27.94,138.43 27.94,121.28 26.67,120.02 20.42,120.02 K1.A2 19.4,120.94 22.23,118.11 22.23,103.5 20.64,101.92 | 20.64,101.92 D2.A | Q1.C 17.78,99.06 20.64,101.92
N$14
  Bottom 0.813: L12.A 7.62,31.11 RL12.2
N$15
  Bottom 0.813: OK3.1 180.34,106.68 D1.C
N$16
  Bottom 0.813: OK3.2 182.88,104.14 R1.1
N$17  (via drill 1 pad 2.03)
  other vias: 68.58,76.83
N$18
  Bottom 0.813: OK3.4 179.71,116.84 177.16,119.38 D4.C
N$19
  Bottom 0.813: RLI1.1 146.05,123.83 R12.2 142.88,118.75 C3.+ 139.06,109.86 R11.1 142.24,104.78 142.88,104.14 142.88,102.87 140.97,100.97 OK6.1
N$20
  Bottom 0.813: D7.C R12.1
N$21
  Bottom 0.813: RLI2.1 110.49,123.83 R14.2 113.03,120.65 C4.+ 116.84,110.49 R13.1 113.03,106.05 OK7.1
N$22
  Bottom 0.813: D8.C R14.1
N$23
  Bottom 0.813: L5.A RL5.1
N$24
  Bottom 0.813: LI2.A RLI2.2
N$25  (via drill 1 pad 2.03)
  Bottom 0.406: U1.16 155.85,54.34 157.48,52.7 157.48,30.48 CA4.+
  Bottom 0.813: U1.16 153.67,54.34 152.4,55.6 v152.4,71.12
N$26
  Bottom 0.813: OK10.1 166.37,106.68 168.28,104.78 D13.C
N$27
  Bottom 0.813: OK10.2 172.37,109.22 175.41,106.81 175.41,103.02 172.72,101.6 R19.1
N$28  (via drill 1 pad 2.03)
  other vias: 66.04,76.83
N$29
  Bottom 0.813: LI1.A 146.05,137.16 146.63,137.22 RLI1.2
N$30
  Bottom 0.813: LO1.K 186.69,134.62 189.87,131.44 R21.1
N$31
  Bottom 0.813: R22.1 158.75,130.81 162.56,134.62 LO2.K
N$32
  Bottom 0.406: RA5.2 66.67,19.84 67.35,19.17 67.35,15.22 S4.2
  Bottom 0.813: RA6.1 131.17,8.61 78.38,8.61 72.98,12.74 | S4.2 72.98,12.74 | 72.98,12.74 S4.1
N$33  (via drill 1 pad 2.03)
  other vias: 139.7,77.47
N$34  (via drill 1 pad 2.03)
  other vias: 142.24,77.47
N$52
  Bottom 0.813: D14.C 161.93,119.38 164.47,116.84 OK10.4
NC1
  Bottom 0.813: K1.NC 33.66,111.09 33.66,133.35 J2.3
NC2
  Bottom 0.813: J3.3 59.69,135.89 62.71,132.87 62.71,110.94 K3.NC
NO1
  Bottom 0.813: J2.1 20.32,133.35 15.88,128.91 15.88,112.36 K1.NO
NO2
  Bottom 0.813: K3.NO 45.09,112.36 45.09,132.08 J3.1
OUT1
  Bottom 0.813: LO1.A 177.76,137.16 DIGITAL-OUT.1 182.88,129.5 OK3.3
OUT2
  Bottom 0.813: LO2.A 170.22,137.16 DIGITAL-OUT.2 171.49,132.75 168.91,130.18 OK10.3
R1  (via drill 1 pad 2.03)
  Top 0.813: v194.31,77.47 194.31,72.39 193.04,71.12 188.7,71.12 162.56,44.98 162.56,33.66 160.38,31.48 U1.25
  Bottom 0.406: U1.25 155.22,31.75
  Bottom 0.813: U1.25 144.15,31.48 v143.51,31.75 | D1.A 194.31,99.06 v194.31,77.47
R2  (via drill 0.9 pad 2.03, 1 pad 2.03)
  Top 0.813: v191.77,77.47 191.77,73.66 191.13,73.03 188.59,73.03 159.38,43.81 v159.38,38.1
  Bottom 0.406: 155.26,28.89 154.94,28.57 | 154.58,28.57 U1.26
  Bottom 0.813: D13.A 156.21,104.78 154.31,102.23 154.31,95.89 156.21,93.98 186.69,93.98 191.77,88.9 v191.77,77.47 | U1.26 154.31,28.57 | 154.94,28.57 154.58,28.57 154.31,28.57 | 154.31,28.57 v143.51,28.57 | U1.26 155.22,28.93 155.26,28.89 | v159.38,38.1 159.38,31.75 165.74,26.04 165.74,24.13 165.1,23.5 160.66,23.5 157.49,26.66 157.49,27.93 156.49,28.93 U1.26
RR1  (via drill 1 pad 2.03)
  Top 0.813: v166.37,70.48 166.37,71.75 173.35,77.47 v176.53,77.47
  Bottom 0.406: U1.3 180.06,24.13
  Bottom 0.813: OK1.1 23.5,83.19 26.67,80.01 174.62,80.01 176.53,78.11 v176.53,77.47 | U1.3 179.53,23.86 166.37,33.84 v166.37,70.48
RR2  (via drill 1 pad 2.03)
  Top 0.813: v168.91,70.48 168.91,71.75 172.91,74.49 177.86,74.49 179.07,75.69 v179.07,77.47
  Bottom 0.406: U1.4 180.7,26.67
  Bottom 0.813: v179.07,77.47 179.07,80.64 177.8,81.92 56.52,81.92 53.34,83.82 OK2.1 | U1.4 179.6,26.39 168.91,34.54 v168.91,70.48
RX0
  Bottom 0.406: U1.12 183.6,46.72 UART.2
RX2
  Bottom 0.406: UART2.2 182.88,29.48 180.88,31.48 U1.6
S1  (via drill 0.9 pad 2.03, 1 pad 2.03)
  Top 0.813: v144.78,71.12 144.78,72.72 146.2,73.51 157.43,73.51 158.12,74.82 v158.12,91.44
  Bottom 0.813: v189.23,77.47 189.23,87.63 185.42,91.44 v158.12,91.44 131.06,91.44 129.54,92.96 R25.2 | v144.78,71.12 144.78,52.7 150.77,46.72 U1.19 | R25.2 129.41,96.65 | OK6.3 133.99,101.6 133.99,99.69 130.81,96.52 129.67,96.52 R25.2
S2  (via drill 1 pad 2.03)
  Top 0.813: v186.69,77.47 186.69,73.66 157.21,44.17 U1.20
  Bottom 0.406: U1.20 154.94,44.45
  Bottom 0.813: v186.69,77.47 186.69,86.36 184.15,88.9 126.36,88.9 125.73,89.53 R26.2 123.19,99.06 OK7.3 | v142.24,71.25 142.24,50.8 148.87,44.17 U1.20
SCK
  Bottom 0.406: U1.9 181.88,39.09 SPI.4
SCL  (via drill 1 pad 2.03)
  Bottom 0.406: U1.14 187.6,51.8 188.59,50.52 I2C.4
  Bottom 0.813: OLED_LCD.3 v100.33,73.03 100.33,75.19 102.87,76.04 173.99,76.04 176.53,73.5 v176.53,70.48 176.53,53.34 178.44,51.44 179.98,51.44 U1.14
SDA  (via drill 1 pad 2.03)  (1 unrouted)
  Bottom 0.406: U1.11 184.51,44.17 186.69,46.35 I2C.3
  Bottom 0.813: OLED_LCD.4 v102.87,73.03 104.14,74.3 142.89,74.3 | U1.11 178.07,44.17 173.99,46.99 v173.99,70.48 173.99,73.03 172.64,74.37 171.65,74.37 171.47,74.39 143.5,74.39 143.51,74.38
TX0
  Bottom 0.406: U1.13 UART.1
TX2
  Bottom 0.406: UART2.1 184.15,33.07 183.52,34.02 U1.7
VN  (via drill 1 pad 2.03)
  Bottom 0.813: v147.32,71.12 147.32,53.34 151.41,49.26 U1.18
VP  (via drill 1 pad 2.03)
  Bottom 0.813: v149.86,71.12 149.86,54.97 153.03,51.8 U1.17
(copper drawn outside any net)
  shapes: Bottom area x112

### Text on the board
Bottom: ISOESP32 VER 0.1 / AGROVOLTAIC / BY ALMUZKY & SALMAN
tPlace: ISOLATION SPACE | CUSTOM SPACE | MICROCONTROLLER | DISPLAY SPACE | POWER DISTRIBUTION | BUTTON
